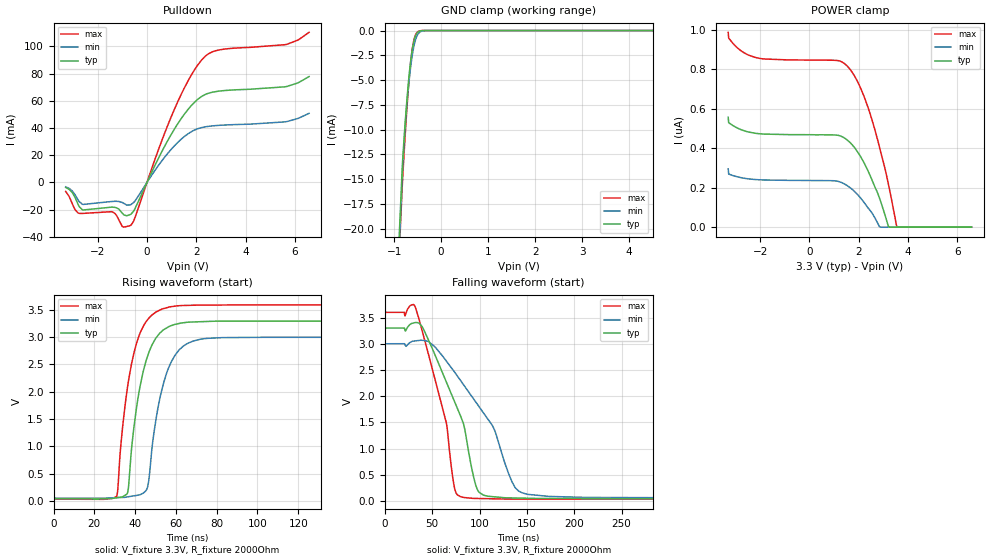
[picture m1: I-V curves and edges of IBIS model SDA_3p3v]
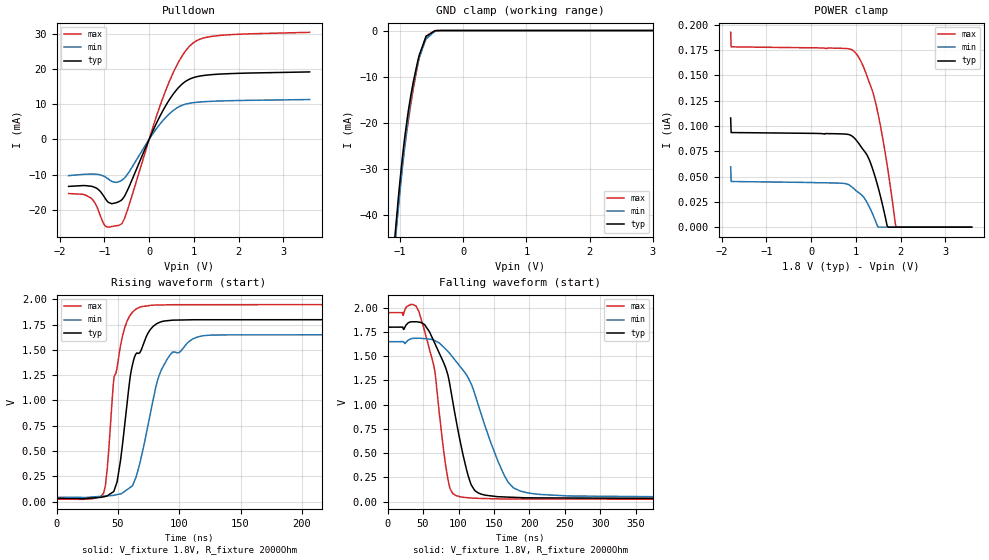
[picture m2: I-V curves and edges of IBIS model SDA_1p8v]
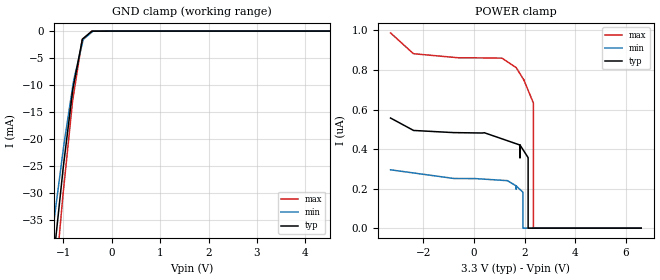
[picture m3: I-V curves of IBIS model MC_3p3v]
|Texas Instruments Incorporated
|2VRMS DIRECTPATH Audio Stereo DAC
| Marketing part#   Voltage Range(Digital)   Package-type   #pins
|PCM5242   1.65V to 3.6V   QFN   32
[IBIS Ver]   4.0
[File name]   pcm5242.ibs
[File Rev]   1.0
[Date]   09/16/2014
[Source]   Texas Instruments Incorporated.
   Analog-eLab, HPA
   12500 TI Blvd
   Dallas, TX -75243
   For Support e-mail: elab_ibis@list.ti.com
[Notes]   Revision History:
   1.0: 09/16/2014
   - Initial version of the model
   - Initial Model generated from simulations.
   - Model names with a trailing _1p8v contains the model for
   1.8V (1.65V and 1.95V). Model names with trailing _3p3v
   contains the model for 3.3V (3.0V and 3.6V) operation.
   - Model not matched to measurements
   - Combined Pulldown/up non-monotonicity warnings for
   GPIO6_xxxx, GPIO_xxxx. LRCK_xxxx and SDA_xxx reflect
   simulation results and can safely ignored.
[Disclaimer]
 This product is designed as an aid for customers of Texas Instruments.
 No warranties, either expressed or implied, with respect to this third
 party software (if any) or with respect to its fitness for any
 particular purpose is claimed by Texas Instruments or the author. The
 software (if any) is provided solely on an "as is" basis. The entire
 risk as to its quality and performance is with the customer
[Copyright] (C) Copyright 2014 Texas Instruments Incorporated.
   All rights reserved.
|   PCM5242
[Component]   pcm5242
[Manufacturer] TI
[Package]   | 32 pin QFN  package
| variable   typ   min   max
R_pkg   0.120   0.037   0.171
L_pkg   1.267nH   0.676nH   1.783nH
C_pkg   0.122pF   0.097pF   0.189pF
|-------------------------PIN------------------------------------------------
[Pin] signal_name  model_name  R_pin  L_pin C_pin
1   XSMT   DEMP_IN   0.14145   1.44228nH   0.11847pF
2   LDOO   TERM   0.11687   1.16108nH   0.10515pF
3   DGND   GND   0.03675   0.67573nH   0.15563pF
4   DVDD   POWER   0.05447   0.73655nH   0.13079pF
5   CPVDD   POWER   0.10887   1.07078nH   0.09677pF
6   CAPP   TERM   0.11363   1.12438nH   0.10023pF
7   CPGND   GND   0.12276   1.22788nH   0.1071pF
8   CAPM   TERM   0.14006   1.42588nH   0.11561pF
9   VNEG   TERM   0.07677   1.15095nH   0.16555pF
10   OUTLP   TERM   0.14272   1.45588nH   0.12303pF
11   OUTLN   TERM   0.12969   1.30498nH   0.11172pF
12   OUTRN   TERM   0.13326   1.34638nH   0.11333pF
13   OUTRP   TERM   0.12721   1.27568nH   0.11024pF
14   AVDD   POWER   0.06367   0.8768nH   0.152pF
15   AGND   GND   0.04389   0.84743nH   0.18869pF
16   VCOM   TERM   0.16265   1.68248nH   0.13615pF
17   SDA/MOSI   SDA   0.17144   1.78348nH   0.1396pF
18   SCL/MC   MC   0.14914   1.52518nH   0.1306pF
19   GPIO5   GPIO   0.12816   1.28348nH   0.11405pF
20   GPIO4   GPIO   0.11696   1.15538nH   0.10388pF
21   GIPIO3   GPIO   0.11201   1.09898nH   0.1001pF
22   ADR2/GPIO2/GPO   GPIO   0.11579   1.14198nH   0.104pF
23   MODE1   MC   0.13014   1.30618nH   0.11523pF
24   MODE2   MC   0.15016   1.53678nH   0.12678pF
25   GPIO6   GPIO   0.1526   1.56608nH   0.12669pF
26   SCK   SCK_IN   0.12814   1.28578nH   0.11005pF
27   BCK   LRCK   0.12793   1.28438nH   0.11056pF
28   DIN   SCK_IN   0.13603   1.37848nH   0.11268pF
29   NC   NC   0.00012   0.00118nH   0.02963pF
30   NC   NC   0.00012   0.00118nH   0.0296pF
31   LRCK   LRCK   0.13176   1.32898nH   0.11078pF
32   ADR1/MISO/FMT   GPIO6   0.1485   1.52258nH   0.12429pF
[Model Selector] SDA
SDA_3p3v   3.3V BCK/LRCK input
SDA_1p8v   1.8V BCK/LRCK input
[Model Selector] GPIO
GPIO_3p3v   3.3V BCK/LRCK input
GPIO_1p8v   1.8V BCK/LRCK input
[Model Selector] GPIO6
GPIO6_3p3v   3.3V BCK/LRCK input
GPIO6_1p8v   1.8V BCK/LRCK input
[Model Selector] LRCK
LRCK_3p3v   3.3V BCK/LRCK input
LRCK_1p8v   1.8V BCK/LRCK input
[Model Selector] MC
MC_3p3v   3.3V BCK/LRCK input
MC_1p8v   1.8V BCK/LRCK input
[Model Selector] DEMP_IN
DEMP_IN_3p3v   3.3V DEMP/SXMT input
DEMP_IN_1p8v   1.8V DEMP/SXMT input
[Model Selector] FLT_IN
FLT_IN_3p3v   3.3V FLT/FMT input
FLT_IN_1p8v   1.8V FLT/FMT input
[Model Selector] SCK_IN
SCK_IN_3p3v   3.3V SCK/DIN input
SCK_IN_1p8v   1.8V SCK/DIN input
[Model Selector] BCK_IN
BCK_IN_3p3v   3.3V BCK/LRCK input
BCK_IN_1p8v   1.8V BCK/LRCK input
|   TERM Model
[Model] TERM
Model_type Terminator
C_comp   0   0   0
| variable   typ   min   max
[Voltage Range]   3.3V   1.65V   3.6V
[POWER Clamp Reference]  3.3V   1.65V   3.6V
[GND Clamp Reference]   0.0V   0.0V   0.0V
|Operating Temperature
[Temperature Range]   27   105   -25
| Models and submodels in the file (19): SDA_3p3v (I/O_open_drain), SDA_1p8v (I/O_open_drain), MC_3p3v (Input), MC_1p8v (Input), LRCK_3p3v (I/O), LRCK_1p8v (I/O), GPIO_3p3v (I/O), GPIO_1p8v (I/O), GPIO6_3p3v (I/O), GPIO6_1p8v (I/O), BCK_IN_1p8v (Input), BCK_IN_3p3v (Input), DEMP_IN_1p8v (Input), DEMP_IN_3p3v (Input), FLT_IN_1p8v (Input), FLT_IN_3p3v (Input), SCK_IN_1p8v (Input), SCK_IN_3p3v (Input), TERM (Terminator)
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|   Model
[Model]   SDA_3p3v
Model_type   I/O_open_drain
Polarity   Non-Inverting
Enable   Active-Low
Vinl = 0.99
Vinh = 2.31
Vmeas = 1.65
Vref = 0
Cref = 1pF
Rref = 1000000
|   typ   min   max
C_comp   1.516pF   1.465pF   1.554pF
[Voltage Range]   3.3   3   3.6
[Temperature Range]   27   105   -25
[Pullup Reference]   3.3   3   3.6
[Pulldown Reference]   -0   -0   -0
[Power Clamp Reference]   3.3   3   3.6
[GND Clamp Reference]   -0   -0   -0
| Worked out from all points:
|   slope of the pulldown table from 0 to 0.495 V, typ, clamps not added: 26.3 ohm
|   GND clamp passes 1 mA (typ) near -0.58 V on its own axis
|   falling waveform, V_fixture 3.3V, R_fixture 2000Ohm: 20-80 % time 34.8ns typ, 52.7ns min, 24.8ns max; typ from 3.3 V to 0.041 V
|   rising waveform, V_fixture 3.3V, R_fixture 2000Ohm: 20-80 % time 8.4ns typ, 8.67ns min, 8.26ns max; typ from 0.041 V to 3.3 V
[Pulldown]
|   Voltage   I(typ)   I(min)   I(max)
-3.3V     -3.69mA    -3.231mA   -6.62mA
-2.924V   -10.89mA   -8.923mA   -19.94mA
-2.627V   -20.05mA   -15.98mA   -22.83mA
-1.439V   -18.19mA   -14.02mA   -21.51mA
-1.003V   -22.57mA   -14.75mA   -32.4mA
-646.8mV  -23.26mA   -16.22mA   -31.41mA
1.115V    39.3mA     26.96mA    53.88mA
1.709V    54.62mA    36.28mA    76.08mA
2.224V    63.3mA     40.35mA    90.14mA
2.917V    67.13mA    41.97mA    97.41mA
5.689V    70.63mA    44.81mA    101.6mA
6.58V     77.86mA    50.82mA    110.4mA
[GND Clamp]
|   Voltage   I(typ)   I(min)   I(max)
-3.3V     -535.5mA   -501.2mA   -563.2mA
-1.003V   -32.53mA   -34.89mA   -33.95mA
-825mV    -13.55mA   -14.3mA    -15.4mA
-785.4mV  -10.63mA   -11.14mA   -12.1mA
-745.8mV  -8.025mA   -8.469mA   -9.073mA
-686.4mV  -4.73mA    -5.259mA   -5.178mA
-646.8mV  -3mA       -3.586mA   -3.142mA
-607.2mV  -1.702mA   -2.273mA   -1.657mA
-567.6mV  -844.6uA   -1.318mA   -738.1uA
-468.6mV  -83.84uA   -220.8uA   -49.26uA
-250.8mV  -157.5nA   -1.094uA   -152.5nA
6.58V     0A         0A         0A
[POWER Clamp]
|   Voltage   I(typ)   I(min)   I(max)
-3.3V     557.1nA    295.8nA    987.7nA
-3.28V    529.8nA    269.3nA    958.9nA
-2.944V   503.4nA    255.7nA    910.8nA
-2.191V   475.9nA    241.3nA    860.1nA
1.432V    451nA      218.1nA    827.9nA
1.947V    382.4nA    165.9nA    738.9nA
2.442V    267.1nA    87.53nA    582nA
2.838V    148.9nA    3.137nA    407.3nA
3.194V    7.28nA     0A         223.6nA
3.531V    0A         0A         8.743nA
3.571V    0A         0A         0A
6.58V     0A         0A         0A
[Ramp]
R_load = 2000
|   typ   min   max
dV/dt_r   1.95361/8.40069e-09   1.76741/8.67093e-09   2.13745/8.26453e-09
dV/dt_f   1.95483/3.47335e-08   1.76784/5.26658e-08   2.13907/2.47647e-08
[Falling Waveform]
V_fixture = 3.3V
V_fixture_min = 3V
V_fixture_max = 3.6V
R_fixture = 2000Ohm
C_fixture = 0F
|   Time   V(typ)   V(min)   V(max)
0s        3.299V     2.999V     3.598V
32.28ns   3.404V     3.054V     3.696V
65.07ns   2.267V     2.668V     1.487V
74.01ns   1.881V     2.452V     218.7mV
79.67ns   1.637V     2.307V     86.41mV
99.44ns   168.7mV    1.802V     48.97mV
116.2ns   80.44mV    1.342V     42.74mV
134.3ns   60.12mV    367.6mV    37.9mV
148.4ns   54.89mV    139.5mV    37.72mV
500ns     40.96mV    53.07mV    33.14mV
[Rising Waveform]
V_fixture = 3.3V
V_fixture_min = 3V
V_fixture_max = 3.6V
R_fixture = 2000Ohm
C_fixture = 0F
|   Time   V(typ)   V(min)   V(max)
0s        40.86mV    52.19mV    33.11mV
31.03ns   59.23mV    60.43mV    85.9mV
35.97ns   125.3mV    72.79mV    2.003V
40.45ns   1.642V     100.3mV    2.851V
44.02ns   2.378V     144.5mV    3.197V
46.62ns   2.706V     352.3mV    3.34V
51.7ns    3.054V     1.8V       3.485V
57.02ns   3.2V       2.487V     3.552V
82.68ns   3.291V     2.989V     3.586V
500ns     3.297V     2.998V     3.596V
|   Model
[Model]   SDA_1p8v
Model_type   I/O_open_drain
Polarity   Non-Inverting
Enable   Active-Low
Vinl = 0.54
Vinh = 1.26
Vmeas = 0.9
Vref = 1.8
Cref = 1pF
Rref = 2000
|   typ   min   max
C_comp   1.609pF   1.569pF   1.650pF
[Voltage Range]   1.8   1.65   1.95
[Temperature Range]   27   105   -25
[Pullup Reference]   1.8   1.65   1.95
[Pulldown Reference]   -0   -0   -0
[Power Clamp Reference]   1.8   1.65   1.95
[GND Clamp Reference]   -0   -0   -0
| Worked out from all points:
|   slope of the pulldown table from 0 to 0.27 V, typ, clamps not added: 37.2 ohm
|   GND clamp passes 1 mA (typ) near -0.56 V on its own axis
|   falling waveform, V_fixture 1.8V, R_fixture 2000Ohm: 20-80 % time 31.3ns typ, 49.5ns min, 21.8ns max; typ from 1.8 V to 0.03 V
|   rising waveform, V_fixture 1.8V, R_fixture 2000Ohm: 20-80 % time 12.2ns typ, 19ns min, 10.6ns max; typ from 0.03 V to 1.8 V
[Pulldown]
|   Voltage   I(typ)   I(min)   I(max)
-1.8V     -13.36mA   -10.29mA   -15.39mA
-1.292V   -13.32mA   -9.837mA   -16.72mA
-979.2mV  -16.82mA   -10.67mA   -24.61mA
-838.8mV  -18.26mA   -11.91mA   -24.78mA
-612mV    -17.19mA   -11.63mA   -23.93mA
-450mV    -13.54mA   -9.314mA   -18.79mA
79.2mV    2.283mA    1.526mA    3.253mA
381.6mV   9.821mA    6.386mA    14.26mA
694.8mV   15.23mA    9.466mA    22.82mA
997.2mV   17.61mA    10.47mA    27.55mA
1.591V    18.59mA    10.94mA    29.59mA
3.589V    19.2mA     11.35mA    30.46mA
[GND Clamp]
|   Voltage   I(typ)   I(min)   I(max)
-1.8V     -178.9mA   -168.7mA   -194.8mA
-1.087V   -45.21mA   -47.13mA   -46.44mA
-1.033V   -36.84mA   -39.13mA   -38.07mA
-979.2mV  -29.3mA    -31.61mA   -30.93mA
-925.2mV  -22.81mA   -24.73mA   -24.89mA
-860.4mV  -16.47mA   -17.59mA   -18.56mA
-795.6mV  -11.35mA   -11.9mA    -12.93mA
-720mV    -6.499mA   -6.967mA   -7.273mA
-698.4mV  -5.332mA   -5.838mA   -5.891mA
-590.4mV  -1.286mA   -1.825mA   -1.201mA
-450mV    -50.58uA   -149.1uA   -26.91uA
3.589V    0A         0A         0A
[POWER Clamp]
|   Voltage   I(typ)   I(min)   I(max)
-1.8V     107.8nA    59.52nA    192.4nA
-1.789V   93.42nA    45.06nA    178.1nA
684mV     92.06nA    43.35nA    176.6nA
943.2mV   88.89nA    38.47nA    174.2nA
1.138V    78nA       31.37nA    161.4nA
1.289V    67.61nA    21.06nA    144.1nA
1.418V    51.37nA    8.308nA    127nA
1.505V    38nA       0A         109.9nA
1.699V    1.187nA    0A         61.12nA
1.883V    0A         0A         2.916nA
1.904V    0A         0A         0A
3.589V    0A         0A         0A
[Ramp]
R_load = 2000
|   typ   min   max
dV/dt_r   1.0613/1.22304e-08   0.964936/1.89179e-08   1.15532/1.06356e-08
dV/dt_f   1.06164/3.11412e-08   0.964359/4.94085e-08   1.15589/2.17745e-08
[Falling Waveform]
V_fixture = 1.8V
V_fixture_min = 1.65V
V_fixture_max = 1.95V
R_fixture = 2000Ohm
C_fixture = 0F
|   Time   V(typ)   V(min)   V(max)
0s        1.8V       1.65V      1.95V
43.65ns   1.853V     1.685V     1.969V
66.47ns   1.634V     1.662V     1.351V
81.83ns   1.383V     1.573V     375mV
88.18ns   1.19V      1.523V     131mV
96.43ns   845.7mV    1.447V     61.72mV
122.8ns   114.5mV    1.113V     34.24mV
164.7ns   47.54mV    266.1mV    26.92mV
186.8ns   40.99mV    108.9mV    26.67mV
500ns     30.38mV    42.62mV    23.13mV
[Rising Waveform]
V_fixture = 1.8V
V_fixture_min = 1.65V
V_fixture_max = 1.95V
R_fixture = 2000Ohm
C_fixture = 0F
|   Time   V(typ)   V(min)   V(max)
0s        30.22mV    41.14mV    23.11mV
38.48ns   46.88mV    53.13mV    84.06mV
41.38ns   56.52mV    55.77mV    330.9mV
46.96ns   108.5mV    62.73mV    1.23V
52.07ns   399.2mV    75.37mV    1.534V
60.94ns   1.298V     147.5mV    1.857V
68.24ns   1.48V      396.9mV    1.923V
85.97ns   1.78V      1.315V     1.944V
118.5ns   1.798V     1.638V     1.947V
500ns     1.799V     1.649V     1.949V
|   Model
[Model]   MC_3p3v
Model_type   Input
Vinl = 0.99
Vinh = 2.31
|   typ   min   max
C_comp   0.996pF   0.979pF   1.002pF
[Voltage Range]   3.3   3   3.6
[Temperature Range]   27   105   -25
[Power Clamp Reference]   3.3   3   3.6
[GND Clamp Reference]   -0   -0   -0
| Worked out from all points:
|   GND clamp passes 1 mA (typ) near -0.54 V on its own axis
[GND Clamp]
|   Voltage   I(typ)   I(min)   I(max)
-3.3V     -526.2mA   -489.4mA   -552.7mA
-1.384V   -58.51mA   -49.12mA   -68.56mA
-1.208V   -42.45mA   -36.01mA   -49.95mA
-1.186V   -40.51mA   -34.34mA   -47.72mA
-1.01V    -25.63mA   -22.28mA   -30.25mA
-806.5mV  -10.7mA    -10.07mA   -12.62mA
-789.9mV  -9.929mA   -9.096mA   -11.67mA
-614.3mV  -1.741mA   -2.396mA   -1.619mA
-591.9mV  -1.35mA    -1.541mA   -1.436mA
-416.3mV  -55.48uA   -203.6uA   -6.973uA
-195.9mV  -8.44uA    -191.8nA   -120.7nA
6.6V      0A         0A         0A
[POWER Clamp]
|   Voltage   I(typ)   I(min)   I(max)
-3.3V     557nA      295.1nA    987.6nA
1.664V    426.9nA    213.3nA    811.6nA
1.926V    398nA      182.2nA    757.5nA
1.927V    397.7nA    0A         757.2nA
2.133V    356.8nA    0A         697.4nA
2.133V    323.7nA    0A         697.3nA
2.134V    0A         0A         697.2nA
2.341V    0A         0A         631.6nA
2.342V    0A         0A         593.6nA
2.342V    0A         0A         422.9nA
2.342V    0A         0A         0A
6.6V      0A         0A         0A
